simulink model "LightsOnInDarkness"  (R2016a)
settings: Solver=FixedStepAuto  StartTime=0.0  StopTime=inf  RelTol=1e-3
libraries: miniQ x2

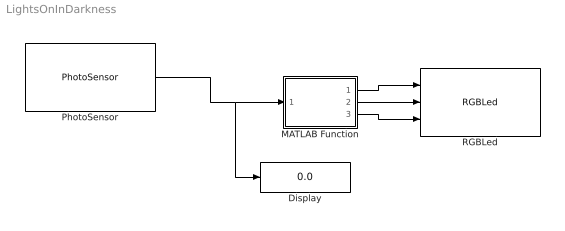
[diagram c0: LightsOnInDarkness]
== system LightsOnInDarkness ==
  Display : Display
  MATLAB Function : MATLAB Function  TreatAsAtomicUnit=on
  PhotoSensor : miniQ/PhotoSensor  sampleTime_dd=0.01  debug_dd=off
  RGBLed : miniQ/RGBLed
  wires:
  PhotoSensor/1 -> Display/1, MATLAB Function/1(lite)
  MATLAB Function/1(red) -> RGBLed/1
  MATLAB Function/2(green) -> RGBLed/2
  MATLAB Function/3(blue) -> RGBLed/3

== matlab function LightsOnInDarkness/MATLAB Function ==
function [red,green,blue] = fcn(lite)

if lite>970
    red=255;
    green=0;
    blue=0;
else
    red=0;
    green=0;
    blue=255;
end
